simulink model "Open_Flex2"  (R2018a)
settings: Solver=VariableStepAuto  StartTime=0.0  StopTime=20.0  RelTol=1e-3
undefined symbols (not defined in the file or in its folder): Ao, Bo, Co, Do

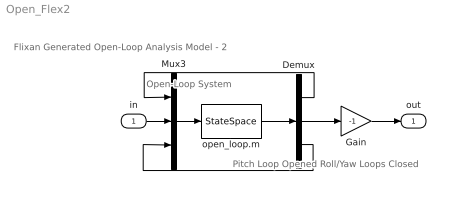
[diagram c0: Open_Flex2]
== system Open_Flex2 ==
  note: Open-Loop System
  note: Pitch Loop Opened Roll/Yaw Loops Closed
  note: Flixan Generated Open-Loop Analysis Model - 2
  in : Inport
  Demux : Demux  Outputs=3
  Gain : Gain  Gain=-1
  Mux3 : Mux  Inputs=3
  open_loop.m : StateSpace  A=Ao  B=Bo  C=Co  D=Do  InitialCondition=0
  out : Outport
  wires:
  Mux3/1 -> open_loop.m/1
  open_loop.m/1 -> Demux/1
  Gain/1 -> out/1
  Demux/3 -> Mux3/3
  in/1 -> Mux3/2
  Demux/2 -> Gain/1
  Demux/1 -> Mux3/1
